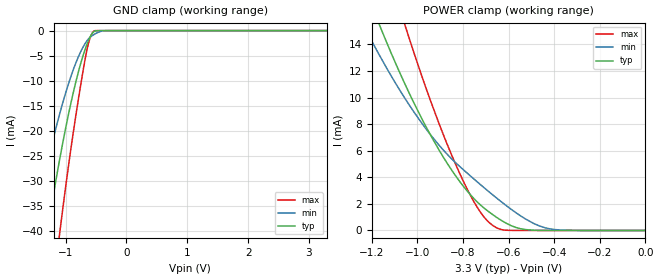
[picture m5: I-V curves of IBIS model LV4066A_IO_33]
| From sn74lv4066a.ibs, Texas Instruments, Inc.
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[Model]   LV4066A_IO_33
Model_type  Terminator
| variable   typ   min   max
C_comp   6.74pF   5.74pF   7.32pF
| C_tri-state   6.74pF   5.74pF   7.32pF
[Temperature Range]   40   100   -40
| Ambient temperature   25   85   -40
[Voltage range]   3.3   3   3.6
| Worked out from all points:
|   GND clamp passes 1 mA (typ) near -0.59 V on its own axis
|   POWER clamp passes 1 mA (typ) near -0.65 V on its own axis
[GND Clamp]
| LV4066A_IO_33
|   Voltage   I(typ)   I(min)   I(max)
-3.3V     -241.7mA   -171.4mA   -346.3mA
-1.535V   -58.89mA   -39.7mA    -88.59mA
-1.315V   -41.17mA   -27.27mA   -63.09mA
-1.28V    -38.52mA   -25.43mA   -59.25mA
-1.11V    -26.47mA   -17.15mA   -41.62mA
-1.08V    -24.49mA   -15.81mA   -38.7mA
-885mV    -12.92mA   -8.155mA   -21.18mA
-685mV    -3.914mA   -2.681mA   -6.021mA
-605mV    -1.447mA   -1.401mA   -1.718mA
-525mV    -116.7uA   -717.4uA   -33.11uA
-300mV    -44.27nA   -5.609uA   -1.9nA
3.3V      81.18pA    3.758uA    60.04pA
[POWER Clamp]
| LV4066A_IO_33
|   Voltage   I(typ)   I(min)   I(max)
-3.3V     163.2mA    126.8mA    216.6mA
-1.255V   19.35mA    16.05mA    27.28mA
-1.215V   17.54mA    14.72mA    24.76mA
-1.175V   15.81mA    13.44mA    22.31mA
-1.135V   14.14mA    12.21mA    19.95mA
-1.055V   11.02mA    9.938mA    15.45mA
-815mV    3.692mA    4.819mA    4.301mA
-740mV    2.183mA    3.689mA    1.804mA
-675mV    1.255mA    2.75mA     445.9uA
-570mV    236.3uA    1.36mA     2.957uA
-440mV    3.205uA    202.1uA    16.12nA
-48.03fV  81.18pA    600.9pA    82.84pA
